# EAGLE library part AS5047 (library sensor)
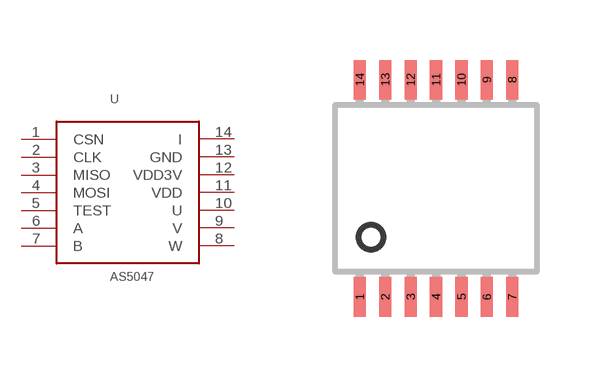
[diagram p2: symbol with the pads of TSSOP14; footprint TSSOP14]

Designator prefix U

## AS5047  [TSSOP14]
1  CSN
2  CLK
3  MISO
4  MOSI
5  TEST
6  A
7  B
8  W
9  V
10  U
11  VDD
12  VDD3V
13  GND
14  I

## Footprint TSSOP14 (pad centres in mm)
Thin Shrink Small Outline Plastic 14
smd 0.305 x 0.991: 1 -1.905,-2.718; 2 -1.27,-2.718; 3 -0.635,-2.718; 4 0,-2.718; 5 0.635,-2.718; 6 1.27,-2.718; 7 1.905,-2.718; 8 1.905,2.718; 9 1.27,2.718; 10 0.635,2.718; 11 0,2.718; 12 -0.635,2.718; 13 -1.27,2.718; 14 -1.905,2.718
